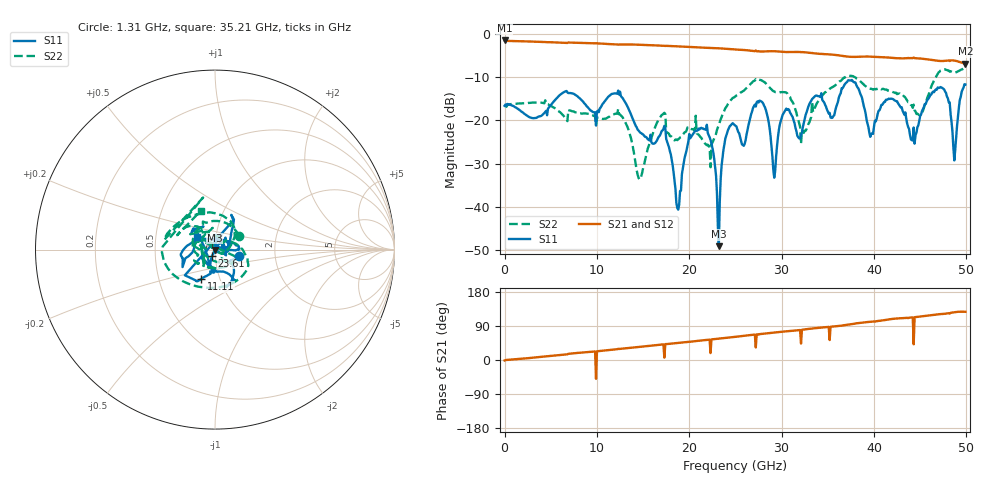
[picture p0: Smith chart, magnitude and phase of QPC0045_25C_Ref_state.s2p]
!File name = QPC0045_25C_Ref_State.s2p
!Date Time: 2024/05/02 05:42:16 AM
!Cal Ref Plane:TRL
!TEMP = 25C
!Vdd(V) = 3.15
!Vss(V) = 0.000
# GHz  S  DB  R  50
!%	Freq(GHz)  S11(dB)  S11(deg)  S21(dB)  S21(deg)  S12(dB)  S12(deg)  S22(dB)  S22(deg)
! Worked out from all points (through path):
!   500 points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, 10 MHz to 49.91 GHz, reference 50 ohm
!   highest |S21| = -1.58 dB at 10 MHz (marker M1); lowest = -6.9 dB at 49.91 GHz (marker M2)
!   lowest |S11| = -49.0 dB at 23.21 GHz (marker M3), VSWR 1.01, Z = 49.8 - j0.266 ohm
!   |S11| at or under -10 dB: start of sweep to end of sweep
!   |S22| runs from -33.7 to -8.0 dB; largest |S21 - S12| = 0.0023
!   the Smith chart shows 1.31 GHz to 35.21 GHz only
!   S11 on the Smith chart (normalised r, x): 1.31 GHz: 1.31, -0.09; 11.11 GHz: 0.82, -0.28; 23.61 GHz: 0.97, -0.06; 35.21 GHz: 0.81, +0.12
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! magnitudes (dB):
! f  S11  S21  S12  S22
! 10 MHz  -16.7  -1.6  -1.6  -16.7
! 1.31 GHz  -17.2  -1.7  -1.7  -16.2
! 8.41 GHz  -15.5  -2.1  -2.1  -18.5
! 11.11 GHz  -14.9  -2.4  -2.4  -19.4
! 14.61 GHz  -22.6  -2.6  -2.6  -33.7
! 16.71 GHz  -23.8  -2.8  -2.8  -19.7
! 18.81 GHz  -40.6  -3.0  -2.9  -24.4
! 20.01 GHz  -23.2  -3.1  -3.1  -22.0
! 21.81 GHz  -22.2  -3.3  -3.3  -25.6
! 23.21 GHz  -49.0  -3.4  -3.4  -21.0
! 23.61 GHz  -28.7  -3.4  -3.4  -18.7
! 25.01 GHz  -21.2  -3.7  -3.7  -14.5
! 27.81 GHz  -15.7  -4.1  -4.1  -10.7
! 29.21 GHz  -33.2  -4.1  -4.1  -13.3
! 30.31 GHz  -18.0  -4.2  -4.2  -13.5
! 33.31 GHz  -15.1  -4.5  -4.5  -15.7
! 35.21 GHz  -18.3  -4.8  -4.8  -12.8
! 41.61 GHz  -15.0  -5.5  -5.5  -13.1
! 44.21 GHz  -24.7  -5.7  -5.7  -17.1
! 47.41 GHz  -12.5  -6.3  -6.3  -8.3
! 48.71 GHz  -29.3  -6.2  -6.2  -8.9
! 49.91 GHz  -11.7  -6.9  -6.9  -8.1
